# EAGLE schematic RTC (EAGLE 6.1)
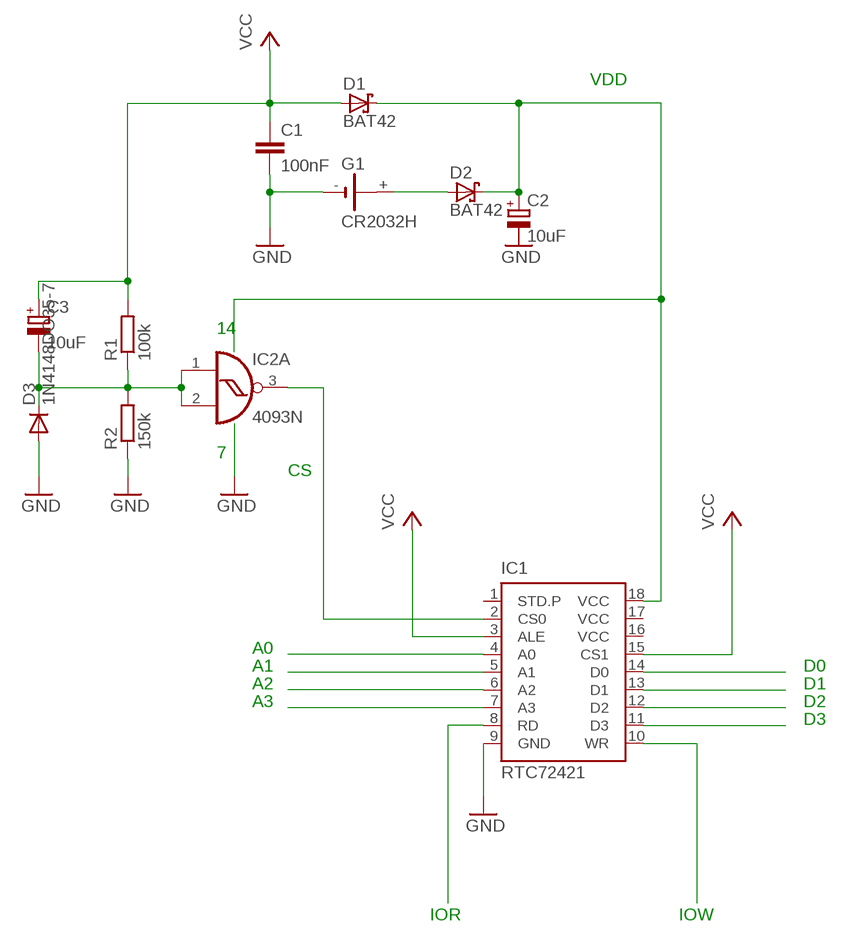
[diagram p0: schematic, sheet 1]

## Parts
C1  100nF  C-EU025-040X050  [C025-040X050]
C2  10uF  CPOL-EU150CLZ-1010  [150CLZ-1010]
C3  10uF  CPOL-EU150CLZ-1010  [150CLZ-1010]
D1  BAT42  [DO35-10]
D2  BAT42  [DO35-10]
D3  1N4148DO35-7  [DO35-7]
G1  CR2032H  [CR2032H]
IC1  RTC72421  [DIL18]
IC2  4093N  [DIL14]
R1  100k  R-EU_0207/7  [0207/7]
R2  150k  R-EU_0207/7  [0207/7]

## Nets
GND: C1.2 D3.A G1.- IC1.9(GND) R2.1
N$1: IC1.10(WR)
N$2: IC1.8(RD)
N$3: IC1.2(CS0) IC2.3(A:O)
N$4: IC1.4(A0)
N$5: IC1.5(A1)
N$6: IC1.6(A2)
N$7: IC1.7(A3)
N$8: IC1.14(D0)
N$9: IC1.13(D1)
N$10: IC1.12(D2)
N$11: IC1.11(D3)
N$12: C2.+ D1.C D2.C IC1.18(VCC)
N$13: D2.A G1.+
N$14: C3.- D3.C IC2.1(A:I0) IC2.2(A:I1) R1.1 R2.2
VCC: C1.1 C3.+ D1.A IC1.3(ALE) IC1.15(CS1) R1.2
Unconnected: C2.- G1.+@1(+) IC1.1(STD.P) IC2.4(B:O) IC2.5(B:I0) IC2.6(B:I1) IC2.8(C:I0) IC2.9(C:I1) IC2.10(C:O) IC2.11(D:O) IC2.12(D:I0) IC2.13(D:I1)

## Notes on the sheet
- VDD
- 14
- 7
- CS
- A0
- A1 | D0
- A2 | D1
- A3 | D2
- D3
- IOR | IOW

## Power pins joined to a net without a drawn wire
VCC: IC1.16(VCC) IC1.17(VCC)
VDD: IC2.14(P:VDD)
VSS: IC2.7(P:VSS)

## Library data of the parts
C1 = rcl:C-EU: CAPACITOR, European symbol
C2 C3 = rcl:CPOL-EU: POLARIZED CAPACITOR, European symbol
D1 D2 = diode:BAT42: DIODE
D3 = diode:1N4148: DIODE
G1 = battery:CR2032H: LI BATTERY Varta
IC1 = fox-electronics:RTC72421: Real Time Clock http://www.foxonline.com/72421.htm; MPN: RTC72421B; OC_FARNELL: 1216228; OC_NEWARK: 01M8738
IC2 = 40xx:4093: Quad 2-input NAND schmitt trigger
R1 R2 = rcl:R-EU_: RESISTOR, European symbol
